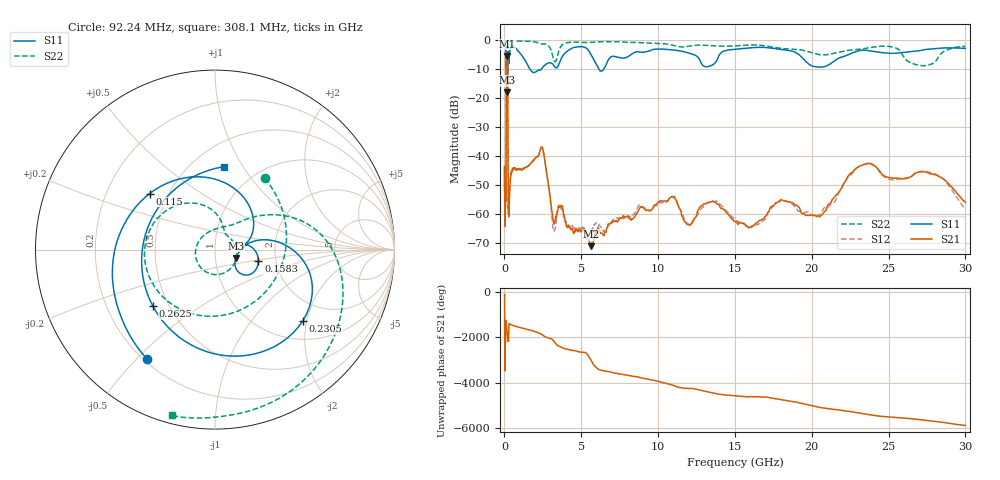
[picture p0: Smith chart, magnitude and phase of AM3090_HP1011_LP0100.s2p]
! Date/Time: Thu, Feb 28, 2019 2:05 PM
! Network Analyzer: Agilent Technologies E8364B Rev: A.07.50.67
! Sweep from 0.010 to 30.000 GHz, 1601 Points, Sweep Type: LOG
! Power Supply: 5.023 V, 0.002 A
# Hz S DB R 50
!freq MagS11 AngS11 MagS21 AngS21 MagS12 AngS12 MagS22 AngS22
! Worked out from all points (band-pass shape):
!   1601 points, 10 MHz to 30 GHz, reference 50 ohm
!   highest |S21| = -5.52 dB at 160.7 MHz (marker M1); lowest = -71.0 dB at 5.64 GHz (marker M2)
!   |S21| within 3 dB of the highest: 129.9 MHz to 200.5 MHz (70.55 MHz wide, 42.7 % of centre)
!   lowest |S11| = -18.0 dB at 190.6 MHz (marker M3), VSWR 1.29, Z = 62.9 - j5.92 ohm
!   |S11| at or under -10 dB: 125.2 MHz to 210.4 MHz (85.2 MHz wide, 50.8 % of centre); 1.649 GHz to 2.393 GHz (744.2 MHz wide, 36.8 % of centre); 6.146 GHz to 6.468 GHz (321.5 MHz wide, 5.1 % of centre)
!   |S22| runs from -20.0 to -0.1 dB; largest |S21 - S12| = 0.013
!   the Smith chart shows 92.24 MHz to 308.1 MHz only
!   S11 on the Smith chart (normalised r, x): 92.24 MHz: 0.21, -0.54; 115 MHz: 0.39, +0.32; 158.3 MHz: 1.62, -0.22; 230.5 MHz: 1.43, -1.89; 262.5 MHz: 0.41, -0.33; 308.1 MHz: 0.70, +0.83
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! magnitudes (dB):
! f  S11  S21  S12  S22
! 10 MHz  -0.2  -46.2  -43.3  -0.5
! 38.04 MHz  -0.4  -60.3  -62.5  -1.3
! 48.61 MHz  -0.7  -52.2  -47.1  -1.4
! 92.24 MHz  -2.9  -54.0  -54.5  -6.3
! 115 MHz  -6.4  -22.7  -22.7  -8.1
! 144.7 MHz  -14.8  -5.9  -5.9  -19.5
! 158.3 MHz  -12.0  -5.5  -5.5  -17.4
! 160.7 MHz  -11.9  -5.5  -5.5  -17.2
! 190.6 MHz  -18.0  -6.7  -6.7  -19.5
! 210.6 MHz  -9.9  -13.9  -13.9  -11.2
! 230.5 MHz  -4.0  -42.9  -42.2  -2.6
! 262.5 MHz  -6.6  -58.0  -56.9  -0.8
! 308.1 MHz  -6.6  -55.3  -58.7  -0.4
! 550.5 MHz  -2.0  -44.4  -44.6  -0.2
! 2.084 GHz  -10.8  -40.4  -40.3  -0.8
! 2.52 GHz  -9.2  -38.1  -38.3  -1.3
! 3.22 GHz  -8.8  -63.3  -65.8  -7.0
! 5.64 GHz  -5.1  -71.0  -66.0  -0.8
! 7.926 GHz  -6.0  -60.9  -61.3  -0.8
! 20.1 GHz  -9.1  -60.4  -60.3  -4.5
! 23.48 GHz  -3.5  -42.7  -42.8  -2.9
! 30 GHz  -2.9  -55.9  -58.3  -2.2
